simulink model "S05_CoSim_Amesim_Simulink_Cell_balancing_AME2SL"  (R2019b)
settings: Solver=ode23s  StartTime=0  StopTime=10000  FixedStep=0.01  RelTol=1e-3  EnableMultiTasking=on
undefined symbols (not defined in the file): S05_CoSim_Amesim_Simulink_Cell_balancing_AME2SL_
libraries: simulink x1
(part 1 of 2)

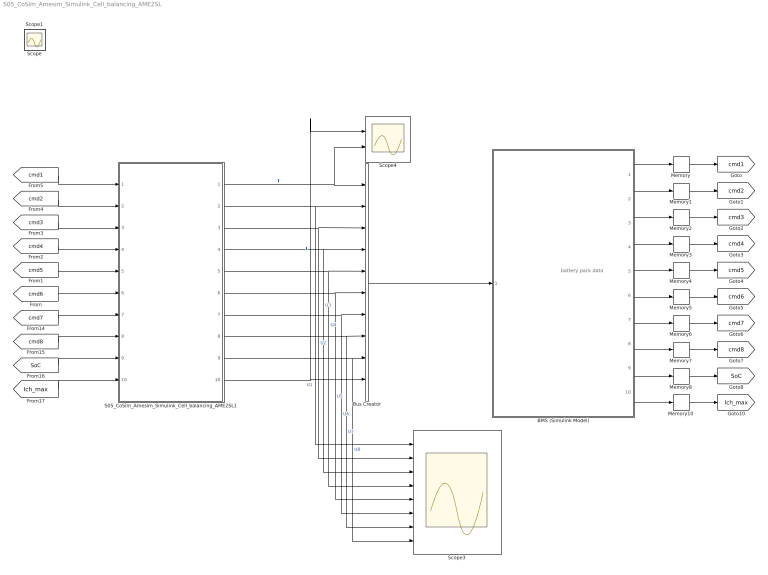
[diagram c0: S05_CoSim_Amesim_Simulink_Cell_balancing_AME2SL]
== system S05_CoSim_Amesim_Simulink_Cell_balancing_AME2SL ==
  note: battery pack data
  " BMS (Simulink Model)" : Subsystem
  Bus Creator : BusCreator  Inputs=10
  Memory{,1..8,10} (10 alike) : Memory
  S05_CoSim_Amesim_Simulink_Cell_balancing_AME2SL1 : Subsystem  Tag=AME2SL  InitFcn=AMESimLib_initBlock  StartFcn=AMESimLib_startBlock  StopFcn=AMESimLib_stopBlock
  Scope3 : Scope  NumInputPorts=8
  Scope4 : Scope  NumInputPorts=2
  Scope : Scope
  Scope1 : Scope
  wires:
  Memory/1 -> [cmd1]
  Memory2/1 -> [cmd3]
  Memory4/1 -> [cmd5]
  Memory3/1 -> [cmd4]
  Memory1/1 -> [cmd2]
  Memory5/1 -> [cmd6]
  Memory6/1 -> [cmd7]
  Memory7/1 -> [cmd8]
  Memory8/1 -> [SoC]
  S05_CoSim_Amesim_Simulink_Cell_balancing_AME2SL1/10(T) -> Scope4/1, Bus Creator/10  "T"
  S05_CoSim_Amesim_Simulink_Cell_balancing_AME2SL1/9(U8) -> Scope3/8, Bus Creator/9  "U8"
  S05_CoSim_Amesim_Simulink_Cell_balancing_AME2SL1/7(U6) -> Scope3/6, Bus Creator/7  "U6"
  S05_CoSim_Amesim_Simulink_Cell_balancing_AME2SL1/6(U5) -> Scope3/5, Bus Creator/6  "U5"
  S05_CoSim_Amesim_Simulink_Cell_balancing_AME2SL1/5(U4) -> Scope3/4, Bus Creator/5  "U4"
  S05_CoSim_Amesim_Simulink_Cell_balancing_AME2SL1/4(U3) -> Scope3/3, Bus Creator/4  "U3"
  S05_CoSim_Amesim_Simulink_Cell_balancing_AME2SL1/3(U2) -> Scope3/2, Bus Creator/3  "U2"
  S05_CoSim_Amesim_Simulink_Cell_balancing_AME2SL1/2(U1) -> Scope3/1, Bus Creator/2  "U1"
  S05_CoSim_Amesim_Simulink_Cell_balancing_AME2SL1/8(U7) -> Scope3/7, Bus Creator/8  "U7"
  [cmd1] -> S05_CoSim_Amesim_Simulink_Cell_balancing_AME2SL1/1(command_cell1)
  [cmd2] -> S05_CoSim_Amesim_Simulink_Cell_balancing_AME2SL1/2(command_cell2)
  [cmd3] -> S05_CoSim_Amesim_Simulink_Cell_balancing_AME2SL1/3(command_cell3)
  [cmd4] -> S05_CoSim_Amesim_Simulink_Cell_balancing_AME2SL1/4(command_cell4)
  [cmd5] -> S05_CoSim_Amesim_Simulink_Cell_balancing_AME2SL1/5(command_cell5)
  [cmd6] -> S05_CoSim_Amesim_Simulink_Cell_balancing_AME2SL1/6(command_cell6)
  [cmd7] -> S05_CoSim_Amesim_Simulink_Cell_balancing_AME2SL1/7(command_cell7)
  [cmd8] -> S05_CoSim_Amesim_Simulink_Cell_balancing_AME2SL1/8(command_cell8)
  [SoC] -> S05_CoSim_Amesim_Simulink_Cell_balancing_AME2SL1/9(SoC)
  S05_CoSim_Amesim_Simulink_Cell_balancing_AME2SL1/1(I) -> Scope4/2, Bus Creator/1  "I"
  [Ich_max] -> S05_CoSim_Amesim_Simulink_Cell_balancing_AME2SL1/10(Ich_max)
  Memory10/1 -> [Ich_max]
  " BMS (Simulink Model)"/10(Ich_max) -> Memory10/1
  " BMS (Simulink Model)"/1(command cell1) -> Memory/1
  " BMS (Simulink Model)"/2(command cell2) -> Memory1/1
  " BMS (Simulink Model)"/3(command cell3) -> Memory2/1
  " BMS (Simulink Model)"/4(command cell4) -> Memory3/1
  " BMS (Simulink Model)"/5(command cell5) -> Memory4/1
  " BMS (Simulink Model)"/6(command cell6) -> Memory5/1
  " BMS (Simulink Model)"/7(command cell7) -> Memory6/1
  " BMS (Simulink Model)"/8(command cell8) -> Memory7/1
  " BMS (Simulink Model)"/9(mean SoC) -> Memory8/1
  Bus Creator/1 -> " BMS (Simulink Model)"/1(battery pack data)

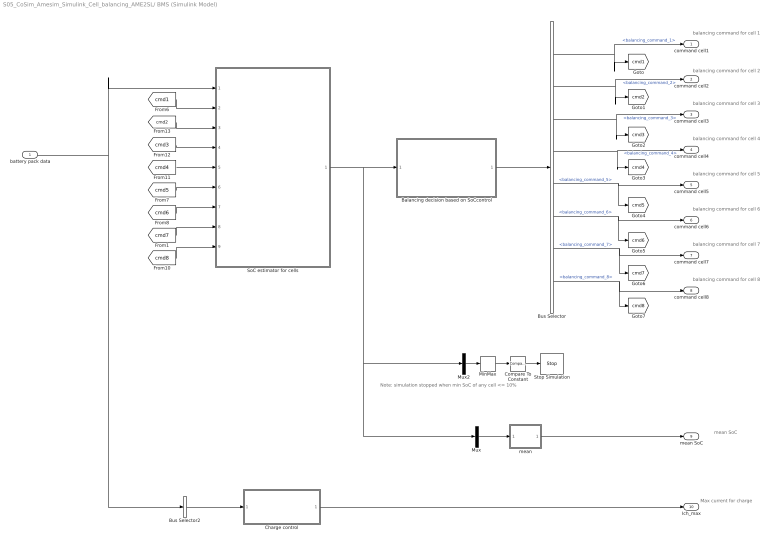
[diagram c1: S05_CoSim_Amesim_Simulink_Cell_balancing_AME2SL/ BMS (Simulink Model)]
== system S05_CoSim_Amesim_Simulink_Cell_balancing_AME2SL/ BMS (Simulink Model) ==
  note: balancing command for cell 1
  note: Max current for charge
  note: mean SoC
  note: Note: simulation stopped when min SoC of any cell <= 10%
  note: balancing command for cell 2
  note: balancing command for cell 3
  note: balancing command for cell 4
  note: balancing command for cell 5
  note: balancing command for cell 6
  note: balancing command for cell 7
  note: balancing command for cell 8
  battery pack data : Inport
  Balancing decision based on SoCcontrol : Subsystem
  Bus Selector : BusSelector  OutputSignals=balancing_command_1,balancing_command_2,balancing_command_3,balancing_command_4,balancing_command_5,balancing_command_6,balancing_command_7,balancing_command_8
  Bus Selector2 : BusSelector  OutputSignals=U1,U2,U3,U4,U5,U6,U7,U8  OutputAsBus=on
  Charge control : Subsystem
  Compare To Constant : simulink/Logic and Bit Operations/Compare To Constant  relop=<=  const=10  OutDataTypeStr=boolean
  MinMax : MinMax
  Mux : Mux  Inputs=1
  Mux2 : Mux  Inputs=1
  SoC estimator for cells : Subsystem
  Stop Simulation : Stop
  mean : MATLAB Function  TreatAsAtomicUnit=on
  command cell1 : Outport
  command cell2 : Outport  Port=2
  command cell3 : Outport  Port=3
  command cell4 : Outport  Port=4
  command cell5 : Outport  Port=5
  command cell6 : Outport  Port=6
  command cell7 : Outport  Port=7
  command cell8 : Outport  Port=8
  mean SoC : Outport  Port=9
  Ich_max : Outport  Port=10
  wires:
  Bus Selector/1 -> [cmd1], command cell1/1  "<balancing_command_1>"
  Bus Selector/6 -> [cmd6], command cell6/1  "<balancing_command_6>"
  Bus Selector/2 -> [cmd2], command cell2/1  "<balancing_command_2>"
  Bus Selector/5 -> [cmd5], command cell5/1  "<balancing_command_5>"
  Bus Selector/4 -> [cmd4], command cell4/1  "<balancing_command_4>"
  Bus Selector/3 -> [cmd3], command cell3/1  "<balancing_command_3>"
  Mux/1 -> mean/1(u)
  Bus Selector/8 -> [cmd8], command cell8/1  "<balancing_command_8>"
  mean/1(y) -> mean SoC/1
  Bus Selector/7 -> [cmd7], command cell7/1  "<balancing_command_7>"
  battery pack data/1 -> Bus Selector2/1, SoC estimator for cells/1(Battery pack data)
  Charge control/1(Ich_max) -> Ich_max/1
  Bus Selector2/1 -> Charge control/1(Ucells)
  Compare To Constant/1 -> Stop Simulation/1
  MinMax/1 -> Compare To Constant/1
  Mux2/1 -> MinMax/1
  Balancing decision based on SoCcontrol/1(balancing_commands) -> Bus Selector/1
  SoC estimator for cells/1(SoCs estimated of cells) -> Mux/1, Mux2/1, Balancing decision based on SoCcontrol/1(SOC_est)
  [cmd1] -> SoC estimator for cells/2(cmd_cell1)
  [cmd2] -> SoC estimator for cells/3(cmd_cell2)
  [cmd3] -> SoC estimator for cells/4(cmd_cell3)
  [cmd4] -> SoC estimator for cells/5(cmd_cell4)
  [cmd6] -> SoC estimator for cells/7(cmd_cell6)
  [cmd7] -> SoC estimator for cells/8(cmd_cell7)
  [cmd8] -> SoC estimator for cells/9(cmd_cell8)
  [cmd5] -> SoC estimator for cells/6(cmd_cell5)

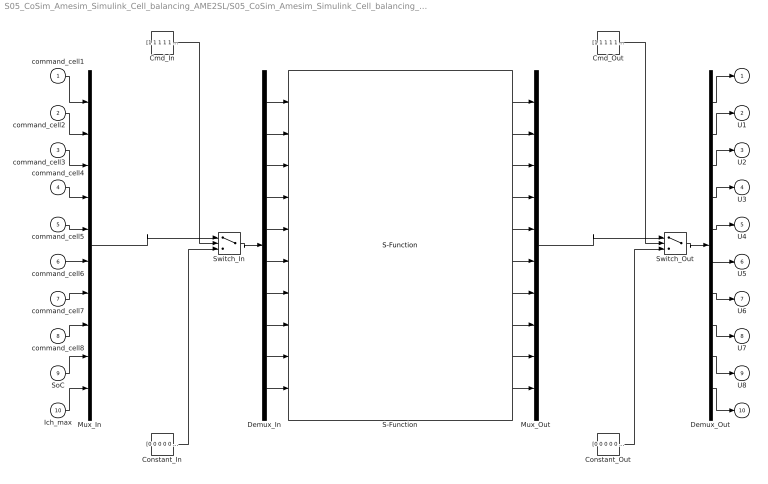
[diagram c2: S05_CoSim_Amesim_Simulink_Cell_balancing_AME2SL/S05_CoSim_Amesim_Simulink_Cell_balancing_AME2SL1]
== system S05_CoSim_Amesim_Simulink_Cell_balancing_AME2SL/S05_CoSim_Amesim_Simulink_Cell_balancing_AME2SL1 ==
  command_cell1 : Inport
  command_cell2 : Inport  Port=2
  command_cell3 : Inport  Port=3
  command_cell4 : Inport  Port=4
  command_cell5 : Inport  Port=5
  command_cell6 : Inport  Port=6
  command_cell7 : Inport  Port=7
  command_cell8 : Inport  Port=8
  SoC : Inport  Port=9
  Ich_max : Inport  Port=10
  Cmd_In : Constant  Value=[1 1 1 1 1 1 1 1 1 1]
  Cmd_Out : Constant  Value=[1 1 1 1 1 1 1 1 1 1]
  Constant_In : Constant  Value=[0 0 0 0 0 0 0 0 0 0]
  Constant_Out : Constant  Value=[0 0 0 0 0 0 0 0 0 0]
  Demux_In : Demux  Outputs=10
  Demux_Out : Demux  Outputs=10
  Mux_In : Mux  Inputs=10
  Mux_Out : Mux  Inputs=10
  S-Function : S-Function  InitFcn=clear S05_CoSim_Amesim_Simulink_Cell_balancing_AME2SL_  StopFcn=clear S05_CoSim_Amesim_Simulink_Cell_balancing_AME2SL_  FunctionName=S05_CoSim_Amesim_Simulink_Cell_balancing_AME2SL_  Parameters="[1,0.01] ['SOCinit      ';'Cn           ';'Ichbalancing ';'Idchbalancing';'Tinit        ';'Tamb         ';'h_cell       ';'w_cell       ';'t_cell       ';'t_plate      ';'t_path       ';'w_path       ';'l_path       ';'DSOC1        ';'DSOC2        ';'DSOC3        ';'DSOC4        ';'DSOC5        ';'DSOC6        ';'DSOC7        ';'DSOC8        ';'Ccoef1       ';'Ccoef2       ';'Ccoef3       ';'Ccoef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"  SFunctionDeploymentMode=off  EnableBusSupport=off
  Switch_In : Switch  Threshold=0.5
  Switch_Out : Switch  Threshold=0.5
  I : Outport
  U1 : Outport  Port=2
  U2 : Outport  Port=3
  U3 : Outport  Port=4
  U4 : Outport  Port=5
  U5 : Outport  Port=6
  U6 : Outport  Port=7
  U7 : Outport  Port=8
  U8 : Outport  Port=9
  T : Outport  Port=10
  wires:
  Mux_In/1 -> Switch_In/1
  Cmd_In/1 -> Switch_In/2
  Constant_In/1 -> Switch_In/3
  Switch_In/1 -> Demux_In/1
  Mux_Out/1 -> Switch_Out/1
  Cmd_Out/1 -> Switch_Out/2
  Constant_Out/1 -> Switch_Out/3
  Switch_Out/1 -> Demux_Out/1
  command_cell1/1 -> Mux_In/1
  Demux_In/1 -> S-Function/1
  command_cell2/1 -> Mux_In/2
  Demux_In/2 -> S-Function/2
  command_cell3/1 -> Mux_In/3
  Demux_In/3 -> S-Function/3
  command_cell4/1 -> Mux_In/4
  Demux_In/4 -> S-Function/4
  command_cell5/1 -> Mux_In/5
  Demux_In/5 -> S-Function/5
  command_cell6/1 -> Mux_In/6
  Demux_In/6 -> S-Function/6
  command_cell7/1 -> Mux_In/7
  Demux_In/7 -> S-Function/7
  command_cell8/1 -> Mux_In/8
  Demux_In/8 -> S-Function/8
  SoC/1 -> Mux_In/9
  Demux_In/9 -> S-Function/9
  Ich_max/1 -> Mux_In/10
  Demux_In/10 -> S-Function/10
  Demux_Out/1 -> I/1
  S-Function/1 -> Mux_Out/1
  Demux_Out/2 -> U1/1
  S-Function/2 -> Mux_Out/2
  Demux_Out/3 -> U2/1
  S-Function/3 -> Mux_Out/3
  Demux_Out/4 -> U3/1
  S-Function/4 -> Mux_Out/4
  Demux_Out/5 -> U4/1
  S-Function/5 -> Mux_Out/5
  Demux_Out/6 -> U5/1
  S-Function/6 -> Mux_Out/6
  Demux_Out/7 -> U6/1
  S-Function/7 -> Mux_Out/7
  Demux_Out/8 -> U7/1
  S-Function/8 -> Mux_Out/8
  Demux_Out/9 -> U8/1
  S-Function/9 -> Mux_Out/9
  Demux_Out/10 -> T/1
  S-Function/10 -> Mux_Out/10

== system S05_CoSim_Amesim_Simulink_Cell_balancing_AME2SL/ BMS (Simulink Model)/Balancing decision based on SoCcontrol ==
  SOC_est : Inport
  Bus Creator1 : BusCreator  Inputs=8
  Bus Selector2 : BusSelector  OutputSignals=SOC1,SOC2,SOC3,SOC4,SOC5,SOC6,SOC7,SOC8
  Bus Selector3 : BusSelector  OutputSignals=SOC1,SOC2,SOC3,SOC4,SOC5,SOC6,SOC7,SOC8
  Mux : Mux  Inputs=8
  Subsystem1 : Subsystem
  Subsystem2 : Subsystem
  Subsystem3 : Subsystem
  Subsystem4 : Subsystem
  Subsystem5 : Subsystem
  Subsystem6 : Subsystem
  Subsystem7 : Subsystem
  Subsystem8 : Subsystem
  median : MATLAB Function  TreatAsAtomicUnit=on
  balancing_commands : Outport
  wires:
  Subsystem1/1(balancing_command) -> Bus Creator1/2  "balancing_command_2"
  Subsystem2/1(balancing_command) -> Bus Creator1/3  "balancing_command_3"
  Subsystem3/1(balancing_command) -> Bus Creator1/4  "balancing_command_4"
  Subsystem4/1(balancing_command) -> Bus Creator1/5  "balancing_command_5"
  Subsystem5/1(balancing_command) -> Bus Creator1/6  "balancing_command_6"
  median/1(y) -> Subsystem8/2(SOC_median), Subsystem7/2(SOC_median), Subsystem5/2(SOC_median), Subsystem4/2(SOC_median), Subsystem3/2(SOC_median), Subsystem2/2(SOC_median), Subsystem1/2(SOC_median), Subsystem6/2(SOC_median)
  Bus Selector2/1 -> Subsystem6/1(SOC_cell)  "<SOC1>"
  Subsystem6/1(balancing_command) -> Bus Creator1/1  "balancing_command_1"
  Bus Selector2/2 -> Subsystem1/1(SOC_cell)  "<SOC2>"
  Bus Selector2/3 -> Subsystem2/1(SOC_cell)  "<SOC3>"
  Bus Selector2/4 -> Subsystem3/1(SOC_cell)  "<SOC4>"
  Bus Selector2/5 -> Subsystem4/1(SOC_cell)  "<SOC5>"
  Bus Selector2/6 -> Subsystem5/1(SOC_cell)  "<SOC6>"
  SOC_est/1 -> Bus Selector3/1, Bus Selector2/1
  Bus Creator1/1 -> balancing_commands/1
  Bus Selector3/1 -> Mux/1  "<SOC1>"
  Bus Selector3/2 -> Mux/2  "<SOC2>"
  Bus Selector3/3 -> Mux/3  "<SOC3>"
  Bus Selector3/4 -> Mux/4  "<SOC4>"
  Bus Selector3/5 -> Mux/5  "<SOC5>"
  Bus Selector3/6 -> Mux/6  "<SOC6>"
  Mux/1 -> median/1(u)
  Bus Selector2/7 -> Subsystem7/1(SOC_cell)  "<SOC7>"
  Bus Selector2/8 -> Subsystem8/1(SOC_cell)  "<SOC8>"
  Subsystem7/1(balancing_command) -> Bus Creator1/7  "balancing_command_7"
  Subsystem8/1(balancing_command) -> Bus Creator1/8  "balancing_command_8"
  Bus Selector3/7 -> Mux/7  "<SOC7>"
  Bus Selector3/8 -> Mux/8  "<SOC8>"

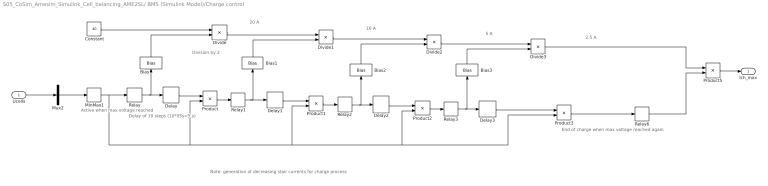
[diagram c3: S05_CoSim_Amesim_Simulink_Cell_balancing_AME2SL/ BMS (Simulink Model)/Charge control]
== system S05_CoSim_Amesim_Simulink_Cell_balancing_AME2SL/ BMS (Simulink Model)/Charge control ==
  note: Note: generation of decreasing stair currents for charge process
  note: Active when max voltage reached
  note: Delay of 10 steps (10*05s=5 s)
  note: 2.5 A
  note: 5 A
  note: 10 A
  note: 20 A
  note: Division by 2
  note: End of charge when max voltage reached again
  Ucells : Inport
  Bias{,1..3} (4 alike) : Bias  Bias=1
  Constant : Constant  Value=40
  Delay{,1..3} (4 alike) : Delay  DelayLength=10
  Divide{,1..3} (4 alike) : Product  Inputs=*/
  MinMax1 : MinMax  Function=max
  Mux2 : Mux  Inputs=1
  Product{,1..3,5} (5 alike) : Product
  Relay{,1..3} (4 alike) : Relay  OnSwitchValue=4.052  OffSwitchValue=4
  Relay6 : Relay  OnSwitchValue=4.052  OffSwitchValue=3.5  OnOutputValue=0  OffOutputValue=1
  Ich_max : Outport
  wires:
  Product3/1 -> Relay6/1
  Relay6/1 -> Product5/2
  Divide2/1 -> Divide3/1
  Product5/1 -> Ich_max/1
  Divide3/1 -> Product5/1
  Divide1/1 -> Divide2/1
  Relay3/1 -> Delay3/1, Bias3/1
  Product2/1 -> Relay3/1
  Bias2/1 -> Divide2/2
  Bias1/1 -> Divide1/2
  Relay1/1 -> Delay1/1, Bias1/1
  Bias3/1 -> Divide3/2
  Divide/1 -> Divide1/1
  MinMax1/1 -> Relay/1, Product3/2, Product2/2, Product1/2, Product/2
  Ucells/1 -> Mux2/1
  Mux2/1 -> MinMax1/1
  Relay/1 -> Delay/1, Bias/1
  Bias/1 -> Divide/2
  Constant/1 -> Divide/1
  Product/1 -> Relay1/1
  Product1/1 -> Relay2/1
  Delay/1 -> Product/1
  Delay1/1 -> Product1/1
  Delay2/1 -> Product2/1
  Delay3/1 -> Product3/1
  Relay2/1 -> Delay2/1, Bias2/1

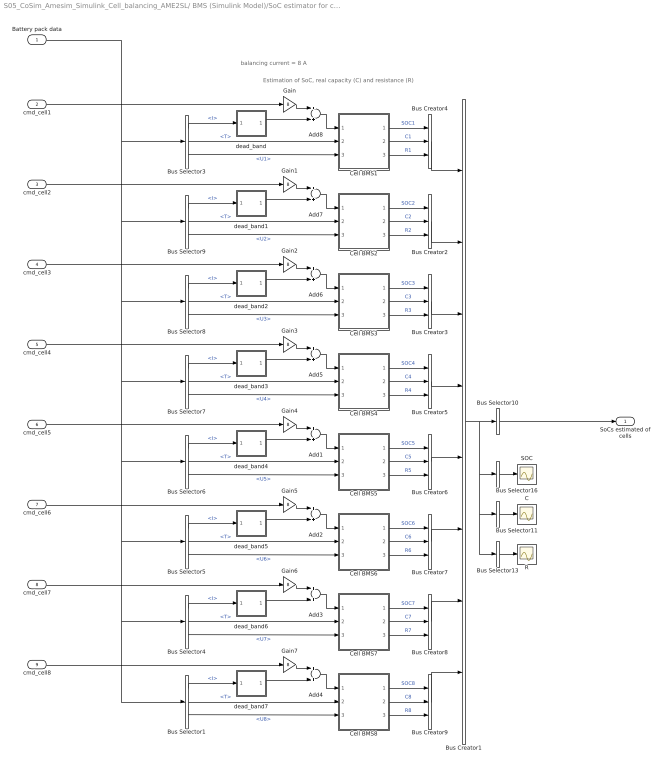
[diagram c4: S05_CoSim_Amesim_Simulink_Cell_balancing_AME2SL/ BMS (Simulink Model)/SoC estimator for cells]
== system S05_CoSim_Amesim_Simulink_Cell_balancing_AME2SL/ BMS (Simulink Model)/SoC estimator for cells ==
  note: Estimation of SoC, real capacity (C) and resistance (R)
  note: balancing current = 8 A
  Battery pack data : Inport
  cmd_cell1 : Inport  Port=2
  cmd_cell2 : Inport  Port=3
  cmd_cell3 : Inport  Port=4
  cmd_cell4 : Inport  Port=5
  cmd_cell5 : Inport  Port=6
  cmd_cell6 : Inport  Port=7
  cmd_cell7 : Inport  Port=8
  cmd_cell8 : Inport  Port=9
  Add{1..8} (8 alike) : Sum
  Bus Creator1 : BusCreator  Inputs=8
  Bus Creator{2..9} (8 alike) : BusCreator  Inputs=3
  Bus Selector1 : BusSelector  OutputSignals=I,T,U8
  Bus Selector10 : BusSelector  OutputSignals=signal1.SOC1,signal2.SOC2,signal3.SOC3,signal4.SOC4,signal5.SOC5,signal6.SOC6,signal7.SOC7,signal8.SOC8  OutputAsBus=on
  Bus Selector11 : BusSelector  OutputSignals=signal1.C1,signal2.C2,signal3.C3,signal4.C4,signal5.C5,signal6.C6,signal7.C7,signal8.C8  OutputAsBus=on
  Bus Selector13 : BusSelector  OutputSignals=signal1.R1,signal2.R2,signal3.R3,signal4.R4,signal5.R5,signal6.R6,signal7.R7,signal8.R8  OutputAsBus=on
  Bus Selector16 : BusSelector  OutputSignals=signal1.SOC1,signal2.SOC2,signal3.SOC3,signal4.SOC4,signal5.SOC5,signal6.SOC6,signal7.SOC7,signal8.SOC8  OutputAsBus=on
  Bus Selector3 : BusSelector  OutputSignals=I,T,U1
  Bus Selector4 : BusSelector  OutputSignals=I,T,U7
  Bus Selector5 : BusSelector  OutputSignals=I,T,U6
  Bus Selector6 : BusSelector  OutputSignals=I,T,U5
  Bus Selector7 : BusSelector  OutputSignals=I,T,U4
  Bus Selector8 : BusSelector  OutputSignals=I,T,U3
  Bus Selector9 : BusSelector  OutputSignals=I,T,U2
  C : Scope
  Cell BMS1 : Subsystem
  Cell BMS2 : Subsystem
  Cell BMS3 : Subsystem
  Cell BMS4 : Subsystem
  Cell BMS5 : Subsystem
  Cell BMS6 : Subsystem
  Cell BMS7 : Subsystem
  Cell BMS8 : Subsystem
  Gain{,1..7} (8 alike) : Gain  Gain=8
  R : Scope
  SOC : Scope
  dead_band : MATLAB Function  TreatAsAtomicUnit=on
  dead_band1 : MATLAB Function  TreatAsAtomicUnit=on
  dead_band2 : MATLAB Function  TreatAsAtomicUnit=on
  dead_band3 : MATLAB Function  TreatAsAtomicUnit=on
  dead_band4 : MATLAB Function  TreatAsAtomicUnit=on
  dead_band5 : MATLAB Function  TreatAsAtomicUnit=on
  dead_band6 : MATLAB Function  TreatAsAtomicUnit=on
  dead_band7 : MATLAB Function  TreatAsAtomicUnit=on
  SoCs estimated of cells : Outport
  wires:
  cmd_cell7/1 -> Gain6/1
  Gain5/1 -> Add2/1
  Bus Creator1/1 -> Bus Selector10/1, Bus Selector16/1, Bus Selector13/1, Bus Selector11/1
  Bus Creator9/1 -> Bus Creator1/8
  Cell BMS7/1(SOC) -> Bus Creator8/1  "SOC7"
  Bus Creator5/1 -> Bus Creator1/4
  Cell BMS8/1(SOC) -> Bus Creator9/1  "SOC8"
  Bus Creator3/1 -> Bus Creator1/3
  Cell BMS5/3(R) -> Bus Creator6/3  "R5"
  Cell BMS3/1(SOC) -> Bus Creator3/1  "SOC3"
  Bus Selector13/1 -> R/1
  Cell BMS4/3(R) -> Bus Creator5/3  "R4"
  Add1/1 -> Cell BMS5/1(I)
  cmd_cell3/1 -> Gain2/1
  Gain/1 -> Add8/1
  Gain3/1 -> Add5/1
  cmd_cell8/1 -> Gain7/1
  cmd_cell5/1 -> Gain4/1
  cmd_cell4/1 -> Gain3/1
  Add2/1 -> Cell BMS6/1(I)
  Gain2/1 -> Add6/1
  Gain1/1 -> Add7/1
  cmd_cell2/1 -> Gain1/1
  Bus Selector16/1 -> SOC/1
  Bus Selector10/1 -> SoCs estimated of cells/1
  Bus Selector11/1 -> C/1
  Cell BMS6/3(R) -> Bus Creator7/3  "R6"
  Cell BMS3/3(R) -> Bus Creator3/3  "R3"
  cmd_cell1/1 -> Gain/1
  Bus Selector3/3 -> Cell BMS1/3(U)  "<U1>"
  Bus Selector1/2 -> Cell BMS8/2(Temp)  "<T>"
  Bus Selector1/3 -> Cell BMS8/3(U)  "<U8>"
  Add8/1 -> Cell BMS1/1(I)
  Bus Selector3/2 -> Cell BMS1/2(Temp)  "<T>"
  Cell BMS3/2(C) -> Bus Creator3/2  "C3"
  Bus Selector1/1 -> dead_band7/1(u)  "<I>"
  Bus Selector4/1 -> dead_band6/1(u)  "<I>"
  Bus Selector7/3 -> Cell BMS4/3(U)  "<U4>"
  Bus Selector5/3 -> Cell BMS6/3(U)  "<U6>"
  Add6/1 -> Cell BMS3/1(I)
  Cell BMS1/3(R) -> Bus Creator4/3  "R1"
  Bus Selector5/2 -> Cell BMS6/2(Temp)  "<T>"
  Bus Selector6/2 -> Cell BMS5/2(Temp)  "<T>"
  Bus Selector9/2 -> Cell BMS2/2(Temp)  "<T>"
  Bus Selector4/2 -> Cell BMS7/2(Temp)  "<T>"
  Add5/1 -> Cell BMS4/1(I)
  Bus Selector7/1 -> dead_band3/1(u)  "<I>"
  Bus Selector5/1 -> dead_band5/1(u)  "<I>"
  Bus Selector4/3 -> Cell BMS7/3(U)  "<U7>"
  Bus Selector6/3 -> Cell BMS5/3(U)  "<U5>"
  Bus Selector8/3 -> Cell BMS3/3(U)  "<U3>"
  Bus Selector7/2 -> Cell BMS4/2(Temp)  "<T>"
  Bus Selector8/1 -> dead_band2/1(u)  "<I>"
  Bus Selector8/2 -> Cell BMS3/2(Temp)  "<T>"
  Bus Selector9/1 -> dead_band1/1(u)  "<I>"
  Cell BMS1/1(SOC) -> Bus Creator4/1  "SOC1"
  Bus Selector9/3 -> Cell BMS2/3(U)  "<U2>"
  Add7/1 -> Cell BMS2/1(I)
  Bus Creator2/1 -> Bus Creator1/2
  Cell BMS2/1(SOC) -> Bus Creator2/1  "SOC2"
  Bus Selector6/1 -> dead_band4/1(u)  "<I>"
  Cell BMS2/3(R) -> Bus Creator2/3  "R2"
  Cell BMS2/2(C) -> Bus Creator2/2  "C2"
  Cell BMS5/1(SOC) -> Bus Creator6/1  "SOC5"
  Cell BMS7/2(C) -> Bus Creator8/2  "C7"
  Cell BMS4/1(SOC) -> Bus Creator5/1  "SOC4"
  Bus Creator6/1 -> Bus Creator1/5
  Cell BMS1/2(C) -> Bus Creator4/2  "C1"
  Bus Creator4/1 -> Bus Creator1/1
  Cell BMS8/3(R) -> Bus Creator9/3  "R8"
  Cell BMS6/1(SOC) -> Bus Creator7/1  "SOC6"
  Cell BMS7/3(R) -> Bus Creator8/3  "R7"
  Cell BMS4/2(C) -> Bus Creator5/2  "C4"
  Cell BMS5/2(C) -> Bus Creator6/2  "C5"
  Bus Creator8/1 -> Bus Creator1/7
  Cell BMS6/2(C) -> Bus Creator7/2  "C6"
  Cell BMS8/2(C) -> Bus Creator9/2  "C8"
  Bus Creator7/1 -> Bus Creator1/6
  Gain6/1 -> Add3/1
  cmd_cell6/1 -> Gain5/1
  Add3/1 -> Cell BMS7/1(I)
  Gain4/1 -> Add1/1
  Add4/1 -> Cell BMS8/1(I)
  Gain7/1 -> Add4/1
  Battery pack data/1 -> Bus Selector1/1, Bus Selector4/1, Bus Selector5/1, Bus Selector6/1, Bus Selector7/1, Bus Selector8/1, Bus Selector9/1, Bus Selector3/1
  dead_band/1(y) -> Add8/2
  Bus Selector3/1 -> dead_band/1(u)  "<I>"
  dead_band1/1(y) -> Add7/2
  dead_band2/1(y) -> Add6/2
  dead_band3/1(y) -> Add5/2
  dead_band4/1(y) -> Add1/2
  dead_band5/1(y) -> Add2/2
  dead_band6/1(y) -> Add3/2
  dead_band7/1(y) -> Add4/2

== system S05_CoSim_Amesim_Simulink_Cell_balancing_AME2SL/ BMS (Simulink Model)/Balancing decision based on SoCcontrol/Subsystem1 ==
  SOC_cell : Inport
  SOC_median : Inport  Port=2
  Add1 : Sum  Inputs=+-
  Add2 : Sum
  Relay : Relay  OnSwitchValue=0.3  OffSwitchValue=0.0  OnOutputValue=-1
  Relay1 : Relay  OnSwitchValue=0.0  OffSwitchValue=-0.3  OnOutputValue=0  OffOutputValue=1
  balancing_command : Outport
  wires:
  SOC_cell/1 -> Add1/1
  SOC_median/1 -> Add1/2
  Add1/1 -> Relay1/1, Relay/1
  Relay1/1 -> Add2/2
  Relay/1 -> Add2/1
  Add2/1 -> balancing_command/1

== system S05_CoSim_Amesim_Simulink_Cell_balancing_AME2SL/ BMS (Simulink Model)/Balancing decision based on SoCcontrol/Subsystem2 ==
  SOC_cell : Inport
  SOC_median : Inport  Port=2
  Add1 : Sum  Inputs=+-
  Add2 : Sum
  Relay : Relay  OnSwitchValue=0.3  OffSwitchValue=0.0  OnOutputValue=-1
  Relay1 : Relay  OnSwitchValue=0.0  OffSwitchValue=-0.3  OnOutputValue=0  OffOutputValue=1
  balancing_command : Outport
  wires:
  SOC_cell/1 -> Add1/1
  SOC_median/1 -> Add1/2
  Add1/1 -> Relay1/1, Relay/1
  Relay1/1 -> Add2/2
  Relay/1 -> Add2/1
  Add2/1 -> balancing_command/1

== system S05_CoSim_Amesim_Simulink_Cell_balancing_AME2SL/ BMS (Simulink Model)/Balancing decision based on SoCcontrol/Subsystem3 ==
  SOC_cell : Inport
  SOC_median : Inport  Port=2
  Add1 : Sum  Inputs=+-
  Add2 : Sum
  Relay : Relay  OnSwitchValue=0.3  OffSwitchValue=0.0  OnOutputValue=-1
  Relay1 : Relay  OnSwitchValue=0.0  OffSwitchValue=-0.3  OnOutputValue=0  OffOutputValue=1
  balancing_command : Outport
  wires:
  SOC_cell/1 -> Add1/1
  SOC_median/1 -> Add1/2
  Add1/1 -> Relay1/1, Relay/1
  Relay1/1 -> Add2/2
  Relay/1 -> Add2/1
  Add2/1 -> balancing_command/1

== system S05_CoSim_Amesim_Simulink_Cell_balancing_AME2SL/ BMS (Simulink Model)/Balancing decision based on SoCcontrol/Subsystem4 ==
  SOC_cell : Inport
  SOC_median : Inport  Port=2
  Add1 : Sum  Inputs=+-
  Add2 : Sum
  Relay : Relay  OnSwitchValue=0.3  OffSwitchValue=0.0  OnOutputValue=-1
  Relay1 : Relay  OnSwitchValue=0.0  OffSwitchValue=-0.3  OnOutputValue=0  OffOutputValue=1
  balancing_command : Outport
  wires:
  SOC_cell/1 -> Add1/1
  SOC_median/1 -> Add1/2
  Add1/1 -> Relay1/1, Relay/1
  Relay1/1 -> Add2/2
  Relay/1 -> Add2/1
  Add2/1 -> balancing_command/1

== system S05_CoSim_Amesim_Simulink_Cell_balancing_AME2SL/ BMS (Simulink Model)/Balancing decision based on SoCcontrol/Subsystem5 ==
  SOC_cell : Inport
  SOC_median : Inport  Port=2
  Add1 : Sum  Inputs=+-
  Add2 : Sum
  Relay : Relay  OnSwitchValue=0.3  OffSwitchValue=0.0  OnOutputValue=-1
  Relay1 : Relay  OnSwitchValue=0.0  OffSwitchValue=-0.3  OnOutputValue=0  OffOutputValue=1
  balancing_command : Outport
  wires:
  SOC_cell/1 -> Add1/1
  SOC_median/1 -> Add1/2
  Add1/1 -> Relay1/1, Relay/1
  Relay1/1 -> Add2/2
  Relay/1 -> Add2/1
  Add2/1 -> balancing_command/1

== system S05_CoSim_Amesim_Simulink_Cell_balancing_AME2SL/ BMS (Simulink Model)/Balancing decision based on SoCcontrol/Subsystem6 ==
  SOC_cell : Inport
  SOC_median : Inport  Port=2
  Add1 : Sum  Inputs=+-
  Add2 : Sum
  Relay : Relay  OnSwitchValue=0.3  OffSwitchValue=0.0  OnOutputValue=-1
  Relay1 : Relay  OnSwitchValue=0.0  OffSwitchValue=-0.3  OnOutputValue=0  OffOutputValue=1
  balancing_command : Outport
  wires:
  SOC_cell/1 -> Add1/1
  SOC_median/1 -> Add1/2
  Add1/1 -> Relay1/1, Relay/1
  Relay1/1 -> Add2/2
  Relay/1 -> Add2/1
  Add2/1 -> balancing_command/1

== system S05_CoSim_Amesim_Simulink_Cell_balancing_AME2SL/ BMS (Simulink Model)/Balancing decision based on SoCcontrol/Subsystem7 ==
  SOC_cell : Inport
  SOC_median : Inport  Port=2
  Add1 : Sum  Inputs=+-
  Add2 : Sum
  Relay : Relay  OnSwitchValue=0.3  OffSwitchValue=0.0  OnOutputValue=-1
  Relay1 : Relay  OnSwitchValue=0.0  OffSwitchValue=-0.3  OnOutputValue=0  OffOutputValue=1
  balancing_command : Outport
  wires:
  SOC_cell/1 -> Add1/1
  SOC_median/1 -> Add1/2
  Add1/1 -> Relay1/1, Relay/1
  Relay1/1 -> Add2/2
  Relay/1 -> Add2/1
  Add2/1 -> balancing_command/1

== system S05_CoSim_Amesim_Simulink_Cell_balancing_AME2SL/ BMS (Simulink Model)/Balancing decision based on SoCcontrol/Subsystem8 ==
  SOC_cell : Inport
  SOC_median : Inport  Port=2
  Add1 : Sum  Inputs=+-
  Add2 : Sum
  Relay : Relay  OnSwitchValue=0.3  OffSwitchValue=0.0  OnOutputValue=-1
  Relay1 : Relay  OnSwitchValue=0.0  OffSwitchValue=-0.3  OnOutputValue=0  OffOutputValue=1
  balancing_command : Outport
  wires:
  SOC_cell/1 -> Add1/1
  SOC_median/1 -> Add1/2
  Add1/1 -> Relay1/1, Relay/1
  Relay1/1 -> Add2/2
  Relay/1 -> Add2/1
  Add2/1 -> balancing_command/1

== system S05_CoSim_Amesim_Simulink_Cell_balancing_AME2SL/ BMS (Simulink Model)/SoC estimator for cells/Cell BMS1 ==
  note: Temperature
  I : Inport
  Temp : Inport  Port=2
  U : Inport  Port=3
  SOC estimator : Subsystem  mask{SOC_init=90, Cnom=42, gainU=50}
      mask prompts: SOC_init "inital state of charge"; Cnom "nominal capacity"; gainU "gain for voltage translation"
  SOH identification : Subsystem
  voltage translation weight : Subsystem
  SOC : Outport
  C : Outport  Port=2
  R : Outport  Port=3
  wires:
  SOC estimator/1(SOC) -> SOC/1
  SOH identification/1(C) -> C/1, SOC estimator/5(C)
  SOC estimator/2(Uerror) -> SOH identification/3(Urerror)
  SOC estimator/3(Icorrect) -> SOH identification/4(Icorrect)
  SOH identification/2(R) -> R/1, SOC estimator/6(R)
  U/1 -> SOC estimator/4(U)
  Temp/1 -> SOC estimator/3(Temp)
  I/1 -> voltage translation weight/1(I), SOC estimator/1(I), SOH identification/1(I)
  voltage translation weight/1(VTweight) -> SOH identification/2(VTweight), SOC estimator/2(VTweight)

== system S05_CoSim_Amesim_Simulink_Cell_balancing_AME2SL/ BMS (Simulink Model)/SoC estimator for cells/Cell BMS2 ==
  I : Inport
  Temp : Inport  Port=2
  U : Inport  Port=3
  SOC estimator : Subsystem  mask{SOC_init=90, Cnom=42, gainU=50}
      mask prompts: SOC_init "inital state of charge"; Cnom "nominal capacity"; gainU "gain for voltage translation"
  SOH identification : Subsystem
  voltage translation weight : Subsystem
  SOC : Outport
  C : Outport  Port=2
  R : Outport  Port=3
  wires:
  SOC estimator/1(SOC) -> SOC/1
  SOH identification/1(C) -> C/1, SOC estimator/5(C)
  SOC estimator/2(Uerror) -> SOH identification/3(Urerror)
  SOC estimator/3(Icorrect) -> SOH identification/4(Icorrect)
  SOH identification/2(R) -> R/1, SOC estimator/6(R)
  U/1 -> SOC estimator/4(U)
  Temp/1 -> SOC estimator/3(Temp)
  I/1 -> voltage translation weight/1(I), SOC estimator/1(I), SOH identification/1(I)
  voltage translation weight/1(VTweight) -> SOH identification/2(VTweight), SOC estimator/2(VTweight)

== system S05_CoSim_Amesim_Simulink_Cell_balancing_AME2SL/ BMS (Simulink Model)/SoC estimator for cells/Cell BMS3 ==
  I : Inport
  Temp : Inport  Port=2
  U : Inport  Port=3
  SOC estimator : Subsystem  mask{SOC_init=90, Cnom=42, gainU=50}
      mask prompts: SOC_init "inital state of charge"; Cnom "nominal capacity"; gainU "gain for voltage translation"
  SOH identification : Subsystem
  voltage translation weight : Subsystem
  SOC : Outport
  C : Outport  Port=2
  R : Outport  Port=3
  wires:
  SOC estimator/1(SOC) -> SOC/1
  SOH identification/1(C) -> C/1, SOC estimator/5(C)
  SOC estimator/2(Uerror) -> SOH identification/3(Urerror)
  SOC estimator/3(Icorrect) -> SOH identification/4(Icorrect)
  SOH identification/2(R) -> R/1, SOC estimator/6(R)
  U/1 -> SOC estimator/4(U)
  Temp/1 -> SOC estimator/3(Temp)
  I/1 -> voltage translation weight/1(I), SOC estimator/1(I), SOH identification/1(I)
  voltage translation weight/1(VTweight) -> SOH identification/2(VTweight), SOC estimator/2(VTweight)

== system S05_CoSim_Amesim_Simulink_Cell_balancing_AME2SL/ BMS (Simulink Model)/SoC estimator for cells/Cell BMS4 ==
  I : Inport
  Temp : Inport  Port=2
  U : Inport  Port=3
  SOC estimator : Subsystem  mask{SOC_init=90, Cnom=42, gainU=50}
      mask prompts: SOC_init "inital state of charge"; Cnom "nominal capacity"; gainU "gain for voltage translation"
  SOH identification : Subsystem
  voltage translation weight : Subsystem
  SOC : Outport
  C : Outport  Port=2
  R : Outport  Port=3
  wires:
  SOC estimator/1(SOC) -> SOC/1
  SOH identification/1(C) -> C/1, SOC estimator/5(C)
  SOC estimator/2(Uerror) -> SOH identification/3(Urerror)
  SOC estimator/3(Icorrect) -> SOH identification/4(Icorrect)
  SOH identification/2(R) -> R/1, SOC estimator/6(R)
  U/1 -> SOC estimator/4(U)
  Temp/1 -> SOC estimator/3(Temp)
  I/1 -> voltage translation weight/1(I), SOC estimator/1(I), SOH identification/1(I)
  voltage translation weight/1(VTweight) -> SOH identification/2(VTweight), SOC estimator/2(VTweight)

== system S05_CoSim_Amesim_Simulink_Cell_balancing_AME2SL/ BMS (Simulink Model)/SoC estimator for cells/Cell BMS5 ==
  I : Inport
  Temp : Inport  Port=2
  U : Inport  Port=3
  SOC estimator : Subsystem  mask{SOC_init=90, Cnom=42, gainU=50}
      mask prompts: SOC_init "inital state of charge"; Cnom "nominal capacity"; gainU "gain for voltage translation"
  SOH identification : Subsystem
  voltage translation weight : Subsystem
  SOC : Outport
  C : Outport  Port=2
  R : Outport  Port=3
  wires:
  SOC estimator/1(SOC) -> SOC/1
  SOH identification/1(C) -> C/1, SOC estimator/5(C)
  SOC estimator/2(Uerror) -> SOH identification/3(Urerror)
  SOC estimator/3(Icorrect) -> SOH identification/4(Icorrect)
  SOH identification/2(R) -> R/1, SOC estimator/6(R)
  U/1 -> SOC estimator/4(U)
  Temp/1 -> SOC estimator/3(Temp)
  I/1 -> voltage translation weight/1(I), SOC estimator/1(I), SOH identification/1(I)
  voltage translation weight/1(VTweight) -> SOH identification/2(VTweight), SOC estimator/2(VTweight)

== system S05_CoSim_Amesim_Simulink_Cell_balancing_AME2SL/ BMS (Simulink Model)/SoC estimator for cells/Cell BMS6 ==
  I : Inport
  Temp : Inport  Port=2
  U : Inport  Port=3
  SOC estimator : Subsystem  mask{SOC_init=90, Cnom=42, gainU=50}
      mask prompts: SOC_init "inital state of charge"; Cnom "nominal capacity"; gainU "gain for voltage translation"
  SOH identification : Subsystem
  voltage translation weight : Subsystem
  SOC : Outport
  C : Outport  Port=2
  R : Outport  Port=3
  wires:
  SOC estimator/1(SOC) -> SOC/1
  SOH identification/1(C) -> C/1, SOC estimator/5(C)
  SOC estimator/2(Uerror) -> SOH identification/3(Urerror)
  SOC estimator/3(Icorrect) -> SOH identification/4(Icorrect)
  SOH identification/2(R) -> R/1, SOC estimator/6(R)
  U/1 -> SOC estimator/4(U)
  Temp/1 -> SOC estimator/3(Temp)
  I/1 -> voltage translation weight/1(I), SOC estimator/1(I), SOH identification/1(I)
  voltage translation weight/1(VTweight) -> SOH identification/2(VTweight), SOC estimator/2(VTweight)

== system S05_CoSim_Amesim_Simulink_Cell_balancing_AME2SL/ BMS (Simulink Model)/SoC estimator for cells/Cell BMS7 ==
  I : Inport
  Temp : Inport  Port=2
  U : Inport  Port=3
  SOC estimator : Subsystem  mask{SOC_init=90, Cnom=42, gainU=50}
      mask prompts: SOC_init "inital state of charge"; Cnom "nominal capacity"; gainU "gain for voltage translation"
  SOH identification : Subsystem
  voltage translation weight : Subsystem
  SOC : Outport
  C : Outport  Port=2
  R : Outport  Port=3
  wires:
  SOC estimator/1(SOC) -> SOC/1
  SOH identification/1(C) -> C/1, SOC estimator/5(C)
  SOC estimator/2(Uerror) -> SOH identification/3(Urerror)
  SOC estimator/3(Icorrect) -> SOH identification/4(Icorrect)
  SOH identification/2(R) -> R/1, SOC estimator/6(R)
  U/1 -> SOC estimator/4(U)
  Temp/1 -> SOC estimator/3(Temp)
  I/1 -> voltage translation weight/1(I), SOC estimator/1(I), SOH identification/1(I)
  voltage translation weight/1(VTweight) -> SOH identification/2(VTweight), SOC estimator/2(VTweight)

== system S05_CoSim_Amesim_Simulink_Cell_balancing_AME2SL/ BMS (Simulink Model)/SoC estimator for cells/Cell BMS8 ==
  I : Inport
  Temp : Inport  Port=2
  U : Inport  Port=3
  SOC estimator : Subsystem  mask{SOC_init=90, Cnom=42, gainU=50}
      mask prompts: SOC_init "inital state of charge"; Cnom "nominal capacity"; gainU "gain for voltage translation"
  SOH identification : Subsystem
  voltage translation weight : Subsystem
  SOC : Outport
  C : Outport  Port=2
  R : Outport  Port=3
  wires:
  SOC estimator/1(SOC) -> SOC/1
  SOH identification/1(C) -> C/1, SOC estimator/5(C)
  SOC estimator/2(Uerror) -> SOH identification/3(Urerror)
  SOC estimator/3(Icorrect) -> SOH identification/4(Icorrect)
  SOH identification/2(R) -> R/1, SOC estimator/6(R)
  U/1 -> SOC estimator/4(U)
  Temp/1 -> SOC estimator/3(Temp)
  I/1 -> voltage translation weight/1(I), SOC estimator/1(I), SOH identification/1(I)
  voltage translation weight/1(VTweight) -> SOH identification/2(VTweight), SOC estimator/2(VTweight)

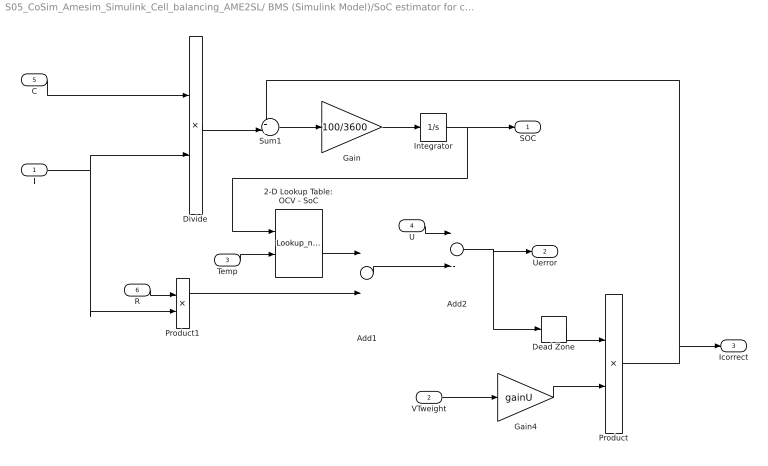
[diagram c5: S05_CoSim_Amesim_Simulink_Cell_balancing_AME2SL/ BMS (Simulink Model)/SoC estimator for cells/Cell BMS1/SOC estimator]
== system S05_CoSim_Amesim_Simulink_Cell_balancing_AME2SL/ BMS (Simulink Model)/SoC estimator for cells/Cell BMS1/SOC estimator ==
  I : Inport
  VTweight : Inport  Port=2
  Temp : Inport  Port=3
  U : Inport  Port=4
  C : Inport  Port=5
  R : Inport  Port=6
  2-D Lookup Table: OCV - SoC : Lookup_n-D  BreakpointsForDimension1=[0, 5, 10, 15, 20, 25, 30, 35, 40, 45, 50, 55, 60, 65, 70, 75, 80, 85, 90, 95, 100]  BreakpointsForDimension2=[0.00, 23.00, 40.00]  Table=[3.00912, 3.025112, 3.036932; 3.332236, 3.339581, 3.34501; 3.459481, 3.463587, 3.466622; 3.495249, 3.49837, 3.500677; 3.531047, 3.53332, 3.535; 3.560502, 3.562569, 3.564097; 3.588662, 3.589579, 3.590256; 3.62715, 3.625996, 3.625143; 3.648255, 3.64543, 3.643341; 3.66652, 3.663455, 3.66119; 3.685242, 3.681938, 3.679495; 3.70967, 3.706246, 3.703715; 3.738426, 3.735163, 3.732751; 3.780458, 3.777286, 3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  InternalRulePriority=Speed  RndMeth=Simplest
  Add1 : Sum
  Add2 : Sum  Inputs=+-
  Dead Zone : DeadZone  LowerValue=-0.005  UpperValue=0.005
  Divide : Product  Inputs=/*
  Gain : Gain  Gain=100/3600
  Gain4 : Gain  Gain=gainU
  Integrator : Integrator  InitialCondition=SOC_init
  Product : Product
  Product1 : Product
  Sum1 : Sum  Inputs=++|
  SOC : Outport
  Uerror : Outport  Port=2
  Icorrect : Outport  Port=3
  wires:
  Integrator/1 -> SOC/1, 2-D Lookup Table: OCV - SoC/1
  Gain/1 -> Integrator/1
  Sum1/1 -> Gain/1
  Add2/1 -> Uerror/1, Dead Zone/1
  Temp/1 -> 2-D Lookup Table: OCV - SoC/2
  C/1 -> Divide/1
  Divide/1 -> Sum1/2
  Gain4/1 -> Product/2
  R/1 -> Product1/1
  2-D Lookup Table: OCV - SoC/1 -> Add1/1
  Add1/1 -> Add2/2
  U/1 -> Add2/1
  Product1/1 -> Add1/2
  I/1 -> Divide/2, Product1/2
  Dead Zone/1 -> Product/1
  Product/1 -> Icorrect/1, Sum1/1
  VTweight/1 -> Gain4/1

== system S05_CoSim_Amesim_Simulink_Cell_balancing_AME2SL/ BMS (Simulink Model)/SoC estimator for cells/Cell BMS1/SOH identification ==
  note: Resistance estimation (ohm)
  note: Capacity estimation (Ah)
  I : Inport
  VTweight : Inport  Port=2
  Urerror : Inport  Port=3
  Icorrect : Inport  Port=4
  Cnom : Constant  Value=42
  Divide : Product  Inputs=**
  Divide1 : Product  Inputs=**
  Integrator3 : Integrator
  Integrator6 : Integrator
  Math Function : Math
  Math Function1 : Math
  Rnom : Constant  Value=0.0022
  Subsystem : Subsystem
  Subsystem6 : Subsystem
  C : Outport
  R : Outport  Port=2
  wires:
  I/1 -> Subsystem6/1(I), Subsystem/1(I)
  Rnom/1 -> Divide1/1
  Divide1/1 -> R/1
  Divide/1 -> C/1
  Subsystem6/1(dCcoef) -> Integrator6/1
  Integrator6/1 -> Math Function/1
  Icorrect/1 -> Subsystem6/3(Icorrect)
  Cnom/1 -> Divide/1
  Urerror/1 -> Subsystem/2(Uerror)
  Subsystem/1(dRcoef) -> Integrator3/1
  Integrator3/1 -> Math Function1/1
  VTweight/1 -> Subsystem6/2(VTweight)
  Math Function/1 -> Divide/2
  Math Function1/1 -> Divide1/2

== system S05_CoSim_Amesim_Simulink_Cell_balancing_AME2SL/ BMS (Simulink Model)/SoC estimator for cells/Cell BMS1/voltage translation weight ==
  I : Inport
  1-D Lookup Table : Lookup_n-D  NumberOfTableDimensions=1  BreakpointsForDimension1=[-0.6,-0.5,-0.1,0,0.1,0.5,0.6]  Table=[0,0,0.2,1,0.2,0,0]  InternalRulePriority=Speed  RndMeth=Simplest
  Add3 : Sum
  Gain2 : Gain  Gain=1/42
  Gain3 : Gain  Gain=0.5
  Transfer Fcn1 : TransferFcn  Denominator=[20*20*20 3*20*20 3*20 1]
  abs : Fcn  Expr=abs(u(1))
  VTweight : Outport
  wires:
  abs/1 -> Transfer Fcn1/1, Add3/1
  Gain2/1 -> abs/1  "Crate"
  Transfer Fcn1/1 -> Add3/2
  Add3/1 -> Gain3/1
  Gain3/1 -> 1-D Lookup Table/1
  I/1 -> Gain2/1
  1-D Lookup Table/1 -> VTweight/1

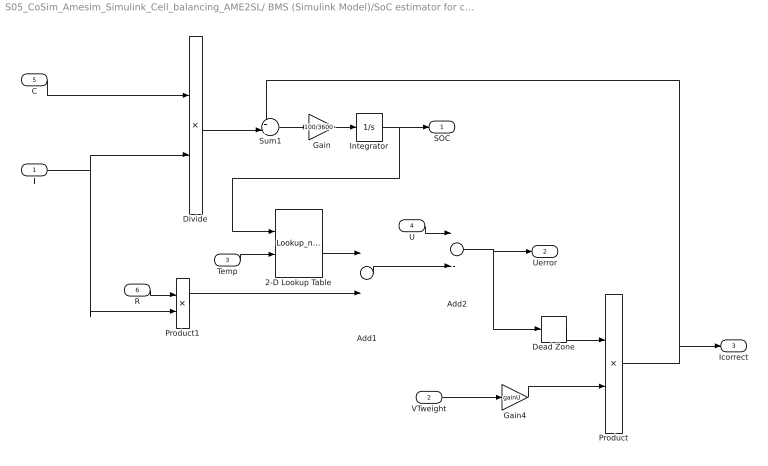
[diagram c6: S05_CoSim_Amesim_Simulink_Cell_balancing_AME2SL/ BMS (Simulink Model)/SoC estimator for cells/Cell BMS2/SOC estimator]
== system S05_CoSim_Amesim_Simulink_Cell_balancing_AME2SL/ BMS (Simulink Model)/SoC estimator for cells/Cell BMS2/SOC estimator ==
  I : Inport
  VTweight : Inport  Port=2
  Temp : Inport  Port=3
  U : Inport  Port=4
  C : Inport  Port=5
  R : Inport  Port=6
  2-D Lookup Table : Lookup_n-D  BreakpointsForDimension1=[0, 5, 10, 15, 20, 25, 30, 35, 40, 45, 50, 55, 60, 65, 70, 75, 80, 85, 90, 95, 100]  BreakpointsForDimension2=[0.00, 23.00, 40.00]  Table=[3.00912, 3.025112, 3.036932; 3.332236, 3.339581, 3.34501; 3.459481, 3.463587, 3.466622; 3.495249, 3.49837, 3.500677; 3.531047, 3.53332, 3.535; 3.560502, 3.562569, 3.564097; 3.588662, 3.589579, 3.590256; 3.62715, 3.625996, 3.625143; 3.648255, 3.64543, 3.643341; 3.66652, 3.663455, 3.66119; 3.685242, 3.681938, 3.679495; 3.70967, 3.706246, 3.703715; 3.738426, 3.735163, 3.732751; 3.780458, 3.777286, 3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  InternalRulePriority=Speed  RndMeth=Simplest
  Add1 : Sum
  Add2 : Sum  Inputs=+-
  Dead Zone : DeadZone  LowerValue=-0.005  UpperValue=0.005
  Divide : Product  Inputs=/*
  Gain : Gain  Gain=100/3600
  Gain4 : Gain  Gain=gainU
  Integrator : Integrator  InitialCondition=SOC_init
  Product : Product
  Product1 : Product
  Sum1 : Sum  Inputs=++|
  SOC : Outport
  Uerror : Outport  Port=2
  Icorrect : Outport  Port=3
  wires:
  Integrator/1 -> SOC/1, 2-D Lookup Table/1
  Gain/1 -> Integrator/1
  Sum1/1 -> Gain/1
  Add2/1 -> Uerror/1, Dead Zone/1
  Temp/1 -> 2-D Lookup Table/2
  C/1 -> Divide/1
  Divide/1 -> Sum1/2
  Gain4/1 -> Product/2
  R/1 -> Product1/1
  2-D Lookup Table/1 -> Add1/1
  Add1/1 -> Add2/2
  U/1 -> Add2/1
  Product1/1 -> Add1/2
  I/1 -> Divide/2, Product1/2
  Dead Zone/1 -> Product/1
  Product/1 -> Icorrect/1, Sum1/1
  VTweight/1 -> Gain4/1

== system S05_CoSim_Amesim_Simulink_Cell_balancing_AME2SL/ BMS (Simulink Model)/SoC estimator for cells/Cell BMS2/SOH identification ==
  I : Inport
  VTweight : Inport  Port=2
  Urerror : Inport  Port=3
  Icorrect : Inport  Port=4
  Cnom : Constant  Value=42
  Divide : Product  Inputs=**
  Divide1 : Product  Inputs=**
  Integrator3 : Integrator
  Integrator6 : Integrator
  Math Function : Math
  Math Function1 : Math
  Rnom : Constant  Value=0.0022
  Subsystem : Subsystem
  Subsystem6 : Subsystem
  C : Outport
  R : Outport  Port=2
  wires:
  I/1 -> Subsystem6/1(I), Subsystem/1(I)
  Rnom/1 -> Divide1/1
  Divide1/1 -> R/1
  Divide/1 -> C/1
  Subsystem6/1(dCcoef) -> Integrator6/1
  Integrator6/1 -> Math Function/1
  Icorrect/1 -> Subsystem6/3(Icorrect)
  Cnom/1 -> Divide/1
  Urerror/1 -> Subsystem/2(Uerror)
  Subsystem/1(dRcoef) -> Integrator3/1
  Integrator3/1 -> Math Function1/1
  VTweight/1 -> Subsystem6/2(VTweight)
  Math Function/1 -> Divide/2
  Math Function1/1 -> Divide1/2

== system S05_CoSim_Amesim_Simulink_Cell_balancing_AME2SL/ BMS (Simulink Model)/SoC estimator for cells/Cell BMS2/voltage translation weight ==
  I : Inport
  1-D Lookup Table : Lookup_n-D  NumberOfTableDimensions=1  BreakpointsForDimension1=[-0.6,-0.5,-0.1,0,0.1,0.5,0.6]  Table=[0,0,0.2,1,0.2,0,0]  InternalRulePriority=Speed  RndMeth=Simplest
  Add3 : Sum
  Gain2 : Gain  Gain=1/42
  Gain3 : Gain  Gain=0.5
  Transfer Fcn1 : TransferFcn  Denominator=[20*20*20 3*20*20 3*20 1]
  abs : Fcn  Expr=abs(u(1))
  VTweight : Outport
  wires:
  abs/1 -> Transfer Fcn1/1, Add3/1
  Gain2/1 -> abs/1  "Crate"
  Transfer Fcn1/1 -> Add3/2
  Add3/1 -> Gain3/1
  Gain3/1 -> 1-D Lookup Table/1
  I/1 -> Gain2/1
  1-D Lookup Table/1 -> VTweight/1

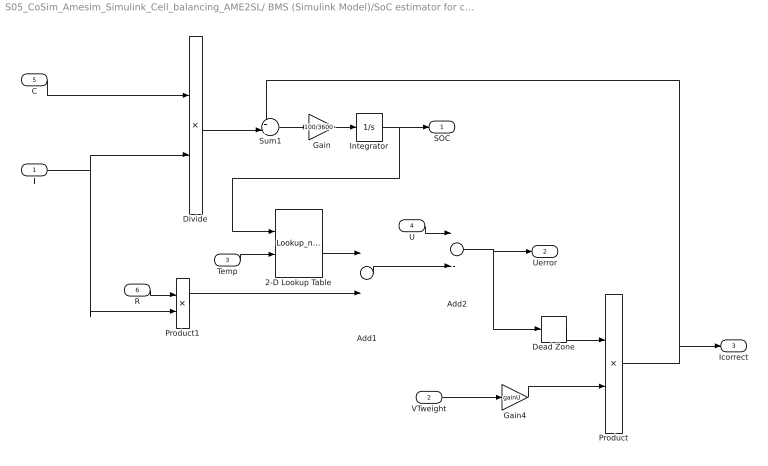
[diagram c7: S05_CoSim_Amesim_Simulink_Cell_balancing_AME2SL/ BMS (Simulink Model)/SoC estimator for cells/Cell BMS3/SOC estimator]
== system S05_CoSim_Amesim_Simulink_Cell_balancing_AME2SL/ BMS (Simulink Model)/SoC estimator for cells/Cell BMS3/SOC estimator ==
  I : Inport
  VTweight : Inport  Port=2
  Temp : Inport  Port=3
  U : Inport  Port=4
  C : Inport  Port=5
  R : Inport  Port=6
  2-D Lookup Table : Lookup_n-D  BreakpointsForDimension1=[0, 5, 10, 15, 20, 25, 30, 35, 40, 45, 50, 55, 60, 65, 70, 75, 80, 85, 90, 95, 100]  BreakpointsForDimension2=[0.00, 23.00, 40.00]  Table=[3.00912, 3.025112, 3.036932; 3.332236, 3.339581, 3.34501; 3.459481, 3.463587, 3.466622; 3.495249, 3.49837, 3.500677; 3.531047, 3.53332, 3.535; 3.560502, 3.562569, 3.564097; 3.588662, 3.589579, 3.590256; 3.62715, 3.625996, 3.625143; 3.648255, 3.64543, 3.643341; 3.66652, 3.663455, 3.66119; 3.685242, 3.681938, 3.679495; 3.70967, 3.706246, 3.703715; 3.738426, 3.735163, 3.732751; 3.780458, 3.777286, 3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  InternalRulePriority=Speed  RndMeth=Simplest
  Add1 : Sum
  Add2 : Sum  Inputs=+-
  Dead Zone : DeadZone  LowerValue=-0.005  UpperValue=0.005
  Divide : Product  Inputs=/*
  Gain : Gain  Gain=100/3600
  Gain4 : Gain  Gain=gainU
  Integrator : Integrator  InitialCondition=SOC_init
  Product : Product
  Product1 : Product
  Sum1 : Sum  Inputs=++|
  SOC : Outport
  Uerror : Outport  Port=2
  Icorrect : Outport  Port=3
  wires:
  Integrator/1 -> SOC/1, 2-D Lookup Table/1
  Gain/1 -> Integrator/1
  Sum1/1 -> Gain/1
  Add2/1 -> Uerror/1, Dead Zone/1
  Temp/1 -> 2-D Lookup Table/2
  C/1 -> Divide/1
  Divide/1 -> Sum1/2
  Gain4/1 -> Product/2
  R/1 -> Product1/1
  2-D Lookup Table/1 -> Add1/1
  Add1/1 -> Add2/2
  U/1 -> Add2/1
  Product1/1 -> Add1/2
  I/1 -> Divide/2, Product1/2
  Dead Zone/1 -> Product/1
  Product/1 -> Icorrect/1, Sum1/1
  VTweight/1 -> Gain4/1

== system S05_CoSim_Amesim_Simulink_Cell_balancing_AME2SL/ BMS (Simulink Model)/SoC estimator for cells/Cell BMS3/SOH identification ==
  I : Inport
  VTweight : Inport  Port=2
  Urerror : Inport  Port=3
  Icorrect : Inport  Port=4
  Cnom : Constant  Value=42
  Divide : Product  Inputs=**
  Divide1 : Product  Inputs=**
  Integrator3 : Integrator
  Integrator6 : Integrator
  Math Function : Math
  Math Function1 : Math
  Rnom : Constant  Value=0.0022
  Subsystem : Subsystem
  Subsystem6 : Subsystem
  C : Outport
  R : Outport  Port=2
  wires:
  I/1 -> Subsystem6/1(I), Subsystem/1(I)
  Rnom/1 -> Divide1/1
  Divide1/1 -> R/1
  Divide/1 -> C/1
  Subsystem6/1(dCcoef) -> Integrator6/1
  Integrator6/1 -> Math Function/1
  Icorrect/1 -> Subsystem6/3(Icorrect)
  Cnom/1 -> Divide/1
  Urerror/1 -> Subsystem/2(Uerror)
  Subsystem/1(dRcoef) -> Integrator3/1
  Integrator3/1 -> Math Function1/1
  VTweight/1 -> Subsystem6/2(VTweight)
  Math Function/1 -> Divide/2
  Math Function1/1 -> Divide1/2

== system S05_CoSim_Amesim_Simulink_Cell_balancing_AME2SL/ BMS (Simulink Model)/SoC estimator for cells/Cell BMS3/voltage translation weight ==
  I : Inport
  1-D Lookup Table : Lookup_n-D  NumberOfTableDimensions=1  BreakpointsForDimension1=[-0.6,-0.5,-0.1,0,0.1,0.5,0.6]  Table=[0,0,0.2,1,0.2,0,0]  InternalRulePriority=Speed  RndMeth=Simplest
  Add3 : Sum
  Gain2 : Gain  Gain=1/42
  Gain3 : Gain  Gain=0.5
  Transfer Fcn1 : TransferFcn  Denominator=[20*20*20 3*20*20 3*20 1]
  abs : Fcn  Expr=abs(u(1))
  VTweight : Outport
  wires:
  abs/1 -> Transfer Fcn1/1, Add3/1
  Gain2/1 -> abs/1  "Crate"
  Transfer Fcn1/1 -> Add3/2
  Add3/1 -> Gain3/1
  Gain3/1 -> 1-D Lookup Table/1
  I/1 -> Gain2/1
  1-D Lookup Table/1 -> VTweight/1

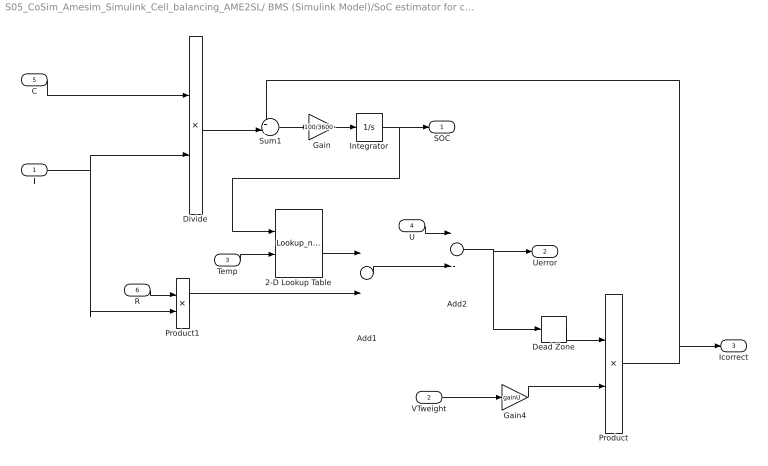
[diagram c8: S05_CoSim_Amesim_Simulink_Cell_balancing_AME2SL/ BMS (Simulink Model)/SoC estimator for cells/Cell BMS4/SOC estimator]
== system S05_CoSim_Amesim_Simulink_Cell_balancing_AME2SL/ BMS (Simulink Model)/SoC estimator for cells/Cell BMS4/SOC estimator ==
  I : Inport
  VTweight : Inport  Port=2
  Temp : Inport  Port=3
  U : Inport  Port=4
  C : Inport  Port=5
  R : Inport  Port=6
  2-D Lookup Table : Lookup_n-D  BreakpointsForDimension1=[0, 5, 10, 15, 20, 25, 30, 35, 40, 45, 50, 55, 60, 65, 70, 75, 80, 85, 90, 95, 100]  BreakpointsForDimension2=[0.00, 23.00, 40.00]  Table=[3.00912, 3.025112, 3.036932; 3.332236, 3.339581, 3.34501; 3.459481, 3.463587, 3.466622; 3.495249, 3.49837, 3.500677; 3.531047, 3.53332, 3.535; 3.560502, 3.562569, 3.564097; 3.588662, 3.589579, 3.590256; 3.62715, 3.625996, 3.625143; 3.648255, 3.64543, 3.643341; 3.66652, 3.663455, 3.66119; 3.685242, 3.681938, 3.679495; 3.70967, 3.706246, 3.703715; 3.738426, 3.735163, 3.732751; 3.780458, 3.777286, 3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  InternalRulePriority=Speed  RndMeth=Simplest
  Add1 : Sum
  Add2 : Sum  Inputs=+-
  Dead Zone : DeadZone  LowerValue=-0.005  UpperValue=0.005
  Divide : Product  Inputs=/*
  Gain : Gain  Gain=100/3600
  Gain4 : Gain  Gain=gainU
  Integrator : Integrator  InitialCondition=SOC_init
  Product : Product
  Product1 : Product
  Sum1 : Sum  Inputs=++|
  SOC : Outport
  Uerror : Outport  Port=2
  Icorrect : Outport  Port=3
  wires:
  Integrator/1 -> SOC/1, 2-D Lookup Table/1
  Gain/1 -> Integrator/1
  Sum1/1 -> Gain/1
  Add2/1 -> Uerror/1, Dead Zone/1
  Temp/1 -> 2-D Lookup Table/2
  C/1 -> Divide/1
  Divide/1 -> Sum1/2
  Gain4/1 -> Product/2
  R/1 -> Product1/1
  2-D Lookup Table/1 -> Add1/1
  Add1/1 -> Add2/2
  U/1 -> Add2/1
  Product1/1 -> Add1/2
  I/1 -> Divide/2, Product1/2
  Dead Zone/1 -> Product/1
  Product/1 -> Icorrect/1, Sum1/1
  VTweight/1 -> Gain4/1

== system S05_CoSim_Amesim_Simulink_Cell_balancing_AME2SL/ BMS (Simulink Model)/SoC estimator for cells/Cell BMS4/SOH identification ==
  I : Inport
  VTweight : Inport  Port=2
  Urerror : Inport  Port=3
  Icorrect : Inport  Port=4
  Cnom : Constant  Value=42
  Divide : Product  Inputs=**
  Divide1 : Product  Inputs=**
  Integrator3 : Integrator
  Integrator6 : Integrator
  Math Function : Math
  Math Function1 : Math
  Rnom : Constant  Value=0.0022
  Subsystem : Subsystem
  Subsystem6 : Subsystem
  C : Outport
  R : Outport  Port=2
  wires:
  I/1 -> Subsystem6/1(I), Subsystem/1(I)
  Rnom/1 -> Divide1/1
  Divide1/1 -> R/1
  Divide/1 -> C/1
  Subsystem6/1(dCcoef) -> Integrator6/1
  Integrator6/1 -> Math Function/1
  Icorrect/1 -> Subsystem6/3(Icorrect)
  Cnom/1 -> Divide/1
  Urerror/1 -> Subsystem/2(Uerror)
  Subsystem/1(dRcoef) -> Integrator3/1
  Integrator3/1 -> Math Function1/1
  VTweight/1 -> Subsystem6/2(VTweight)
  Math Function/1 -> Divide/2
  Math Function1/1 -> Divide1/2

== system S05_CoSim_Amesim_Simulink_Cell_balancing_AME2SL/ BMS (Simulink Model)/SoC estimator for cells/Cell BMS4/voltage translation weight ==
  I : Inport
  1-D Lookup Table : Lookup_n-D  NumberOfTableDimensions=1  BreakpointsForDimension1=[-0.6,-0.5,-0.1,0,0.1,0.5,0.6]  Table=[0,0,0.2,1,0.2,0,0]  InternalRulePriority=Speed  RndMeth=Simplest
  Add3 : Sum
  Gain2 : Gain  Gain=1/42
  Gain3 : Gain  Gain=0.5
  Transfer Fcn1 : TransferFcn  Denominator=[20*20*20 3*20*20 3*20 1]
  abs : Fcn  Expr=abs(u(1))
  VTweight : Outport
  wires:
  abs/1 -> Transfer Fcn1/1, Add3/1
  Gain2/1 -> abs/1  "Crate"
  Transfer Fcn1/1 -> Add3/2
  Add3/1 -> Gain3/1
  Gain3/1 -> 1-D Lookup Table/1
  I/1 -> Gain2/1
  1-D Lookup Table/1 -> VTweight/1

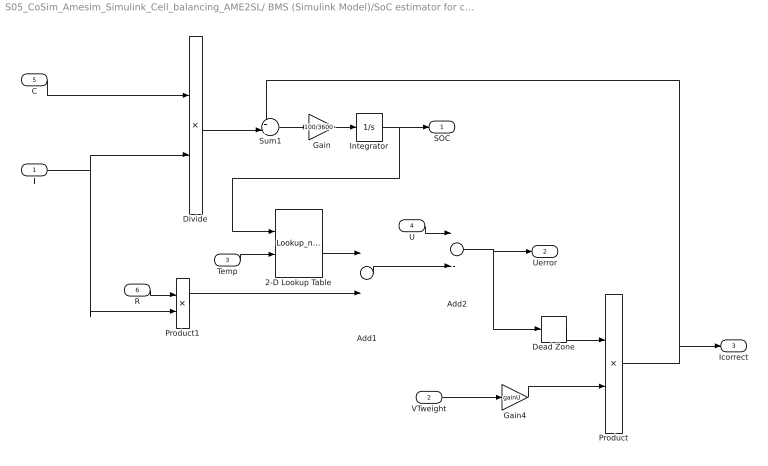
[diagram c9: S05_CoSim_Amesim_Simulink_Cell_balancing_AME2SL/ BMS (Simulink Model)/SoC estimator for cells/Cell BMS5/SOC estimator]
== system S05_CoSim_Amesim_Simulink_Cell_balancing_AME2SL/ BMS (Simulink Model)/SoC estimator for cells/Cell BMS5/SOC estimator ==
  I : Inport
  VTweight : Inport  Port=2
  Temp : Inport  Port=3
  U : Inport  Port=4
  C : Inport  Port=5
  R : Inport  Port=6
  2-D Lookup Table : Lookup_n-D  BreakpointsForDimension1=[0, 5, 10, 15, 20, 25, 30, 35, 40, 45, 50, 55, 60, 65, 70, 75, 80, 85, 90, 95, 100]  BreakpointsForDimension2=[0.00, 23.00, 40.00]  Table=[3.00912, 3.025112, 3.036932; 3.332236, 3.339581, 3.34501; 3.459481, 3.463587, 3.466622; 3.495249, 3.49837, 3.500677; 3.531047, 3.53332, 3.535; 3.560502, 3.562569, 3.564097; 3.588662, 3.589579, 3.590256; 3.62715, 3.625996, 3.625143; 3.648255, 3.64543, 3.643341; 3.66652, 3.663455, 3.66119; 3.685242, 3.681938, 3.679495; 3.70967, 3.706246, 3.703715; 3.738426, 3.735163, 3.732751; 3.780458, 3.777286, 3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  InternalRulePriority=Speed  RndMeth=Simplest
  Add1 : Sum
  Add2 : Sum  Inputs=+-
  Dead Zone : DeadZone  LowerValue=-0.005  UpperValue=0.005
  Divide : Product  Inputs=/*
  Gain : Gain  Gain=100/3600
  Gain4 : Gain  Gain=gainU
  Integrator : Integrator  InitialCondition=SOC_init
  Product : Product
  Product1 : Product
  Sum1 : Sum  Inputs=++|
  SOC : Outport
  Uerror : Outport  Port=2
  Icorrect : Outport  Port=3
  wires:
  Integrator/1 -> SOC/1, 2-D Lookup Table/1
  Gain/1 -> Integrator/1
  Sum1/1 -> Gain/1
  Add2/1 -> Uerror/1, Dead Zone/1
  Temp/1 -> 2-D Lookup Table/2
  C/1 -> Divide/1
  Divide/1 -> Sum1/2
  Gain4/1 -> Product/2
  R/1 -> Product1/1
  2-D Lookup Table/1 -> Add1/1
  Add1/1 -> Add2/2
  U/1 -> Add2/1
  Product1/1 -> Add1/2
  I/1 -> Divide/2, Product1/2
  Dead Zone/1 -> Product/1
  Product/1 -> Icorrect/1, Sum1/1
  VTweight/1 -> Gain4/1

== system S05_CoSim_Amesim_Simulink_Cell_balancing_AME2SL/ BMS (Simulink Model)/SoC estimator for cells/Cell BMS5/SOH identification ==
  I : Inport
  VTweight : Inport  Port=2
  Urerror : Inport  Port=3
  Icorrect : Inport  Port=4
  Cnom : Constant  Value=42
  Divide : Product  Inputs=**
  Divide1 : Product  Inputs=**
  Integrator3 : Integrator
  Integrator6 : Integrator
  Math Function : Math
  Math Function1 : Math
  Rnom : Constant  Value=0.0022
  Subsystem : Subsystem
  Subsystem6 : Subsystem
  C : Outport
  R : Outport  Port=2
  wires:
  I/1 -> Subsystem6/1(I), Subsystem/1(I)
  Rnom/1 -> Divide1/1
  Divide1/1 -> R/1
  Divide/1 -> C/1
  Subsystem6/1(dCcoef) -> Integrator6/1
  Integrator6/1 -> Math Function/1
  Icorrect/1 -> Subsystem6/3(Icorrect)
  Cnom/1 -> Divide/1
  Urerror/1 -> Subsystem/2(Uerror)
  Subsystem/1(dRcoef) -> Integrator3/1
  Integrator3/1 -> Math Function1/1
  VTweight/1 -> Subsystem6/2(VTweight)
  Math Function/1 -> Divide/2
  Math Function1/1 -> Divide1/2
